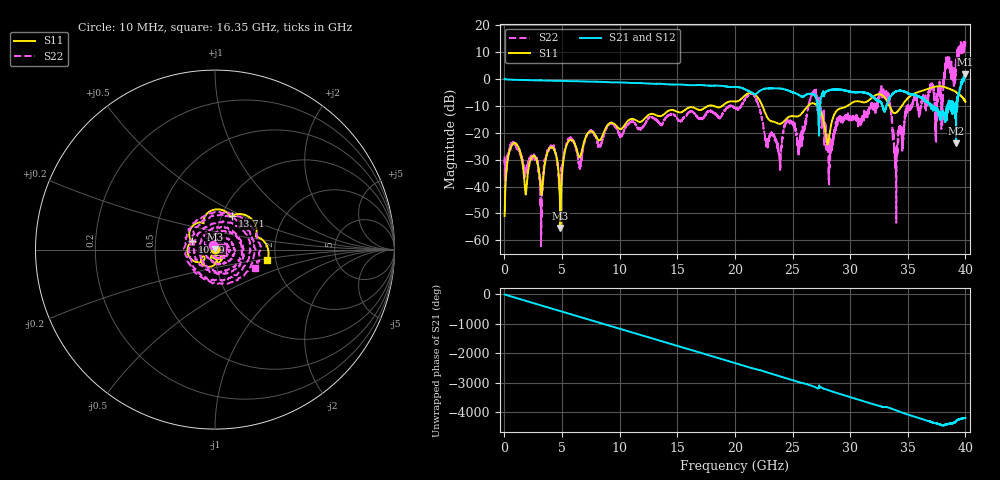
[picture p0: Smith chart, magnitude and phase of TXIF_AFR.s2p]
!Keysight Technologies,N5245B,MY58422297,A.13.80.12
!Automatic Fixture Removal (AFR)
!Date: Tuesday, April 21, 2020, 02:01:44
!S2P File: Measurements: S11,S21,S12,S22:
# MHz S  RI  R 50
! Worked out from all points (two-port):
!   4000 points, 10 MHz to 40 GHz, reference 50 ohm
!   highest |S21| = 1.72 dB at 40 GHz (marker M1); lowest = -24.0 dB at 39.19 GHz (marker M2)
!   |S21| within 3 dB of the highest: start of sweep to 10.12 GHz; 39.68 GHz to end of sweep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
!   lowest |S11| = -55.4 dB at 4.85 GHz (marker M3), VSWR 1.00, Z = 49.9 + j0.141 ohm
!   |S11| at or under -10 dB: start of sweep to 17.67 GHz; 22.38 GHz to 26.33 GHz (3.954 GHz wide, 16.2 % of centre); 27.14 GHz to 29.76 GHz (2.622 GHz wide, 9.22 % of centre)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
!   |S22| runs from -62.2 to 14.3 dB; largest |S21 - S12| = 1e-14
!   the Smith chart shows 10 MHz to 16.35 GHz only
!   S11 on the Smith chart (normalised r, x): 10 MHz: 1.00, +0.01; 10.39 GHz: 0.77, +0.07; 13.71 GHz: 1.12, +0.44; 16.35 GHz: 1.80, -0.24
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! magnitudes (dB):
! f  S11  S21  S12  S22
! 10 MHz  -50.9  0.0  0.0  -31.4
! 850 MHz  -23.8  -0.3  -0.3  -24.2
! 3.18 GHz  -42.3  -0.5  -0.5  -47.3
! 4.19 GHz  -25.5  -0.6  -0.6  -25.1
! 4.85 GHz  -55.4  -0.7  -0.7  -37.6
! 5.53 GHz  -23.3  -0.8  -0.8  -23.0
! 6.68 GHz  -27.4  -0.9  -0.9  -29.5
! 10.39 GHz  -17.4  -1.3  -1.3  -19.1
! 13.34 GHz  -13.8  -1.7  -1.7  -15.8
! 13.71 GHz  -13.5  -1.8  -1.8  -16.6
! 16.35 GHz  -10.5  -2.3  -2.3  -12.2
! 20.01 GHz  -8.4  -2.9  -2.9  -10.8
! 21.58 GHz  -5.4  -5.4  -5.4  -5.6
! 23.87 GHz  -16.7  -3.5  -3.5  -30.7
! 25.63 GHz  -13.5  -6.1  -6.1  -22.8
! 26.67 GHz  -9.0  -5.6  -5.6  -5.7
! 28.21 GHz  -20.5  -4.1  -4.1  -25.7
! 33.34 GHz  -9.4  -7.7  -7.7  -6.1
! 33.98 GHz  -12.6  -4.6  -4.6  -32.2
! 34.96 GHz  -7.3  -5.1  -5.1  -10.5
! 39.19 GHz  -4.8  -24.0  -24.0  4.0
! 40 GHz  -8.4  1.7  1.7  13.9
